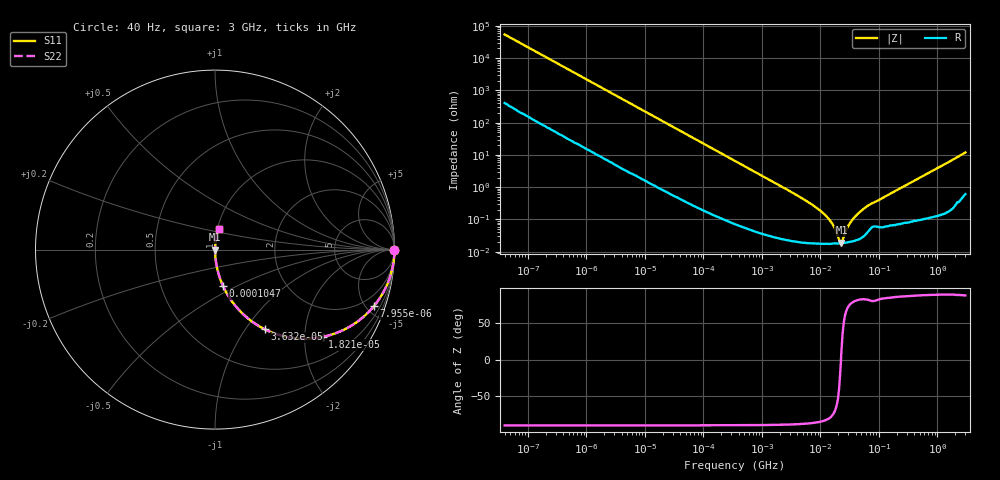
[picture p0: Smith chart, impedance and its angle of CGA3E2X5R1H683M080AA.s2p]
! S-parameter Generated by TDK Corporation
! Copyright(C) 2015 TDK Corporation.
! All Rights Reserved.
! TDK P/N: CGA3E2X5R1H683M080AA (Multilayer Ceramic Chip Capacitors)
! Property: C=68nF
! Size(LxWxT): 1.6x0.8x0.8mm, 0.063x0.031x0.031inches
! Model Type: s2p (Touchstone File Format Version 1.0)
! Frequency: DC=Yes Start=0.00004MHz Stop=3000MHz 396points Log-sweep
! Note: This model was converted from impedance.
! Model Generated on Jun. 23, 2015
! Hash(MD5):
! Port Assignments:
!  1 ---| |--- 2
! Applicable Conditions:
!  Temperature = 25 degC
!  DC Bias Voltage = 0 V
!  Small Signal Operation
! Terms and conditions regarding TDK Simulation Models
! (1)This simulation model is being provided solely for informational purposes. Please refer to the specifications of the products in terms of detailed characteristics of such products.
! (2)In no event shall TDK Corporation of any of its subsidiaries be liable for any loss or damage arising, directly or indirectly,
!  From any information contained in this simulation model, including, but not limited to loss or damages arising from any inaccuracies, omissions or errors in connection with such information.
! (3)Any and all copyrights on this simulation model are owned by TDK Corporation.
!  Duplication or redistribution of this simulation model without prior written permission from TDK Corporation is prohibited.
! (4)This simulation model is subject to any modification or change without any prior notice.
! (5)Neither TDK Corporation nor any of its subsidiaries shall make any warranty, express or implied,
!  Including but not limited to the correctness, implied warranties of merchantability and fitness for a particular purpose with respect to this simulation models.
! (6)The use of this simulation model shall be deemed to have consented to the terms and conditions hereof.
# MHz S MA R 50
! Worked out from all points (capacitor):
!   395 points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, 40 Hz to 3 GHz, reference 50 ohm
!   read as one part in series: C = 73.5 nF near 41.88 Hz
!   lowest |Z| = 19 mohm at 22.83 MHz (marker M1)
!   series resonance near 22.44 MHz, so ESL is about 680 pH
!   S11 on the Smith chart (normalised r, x): 40 Hz: open; 7.955 kHz: 1.04, -5.59; 18.21 kHz: 1.02, -2.45; 36.32 kHz: 1.01, -1.23; 104.7 kHz: 1.00, -0.43; 3 GHz: 1.01, +0.24
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4e-05  1 -0.1  0.001852 89.5  0.001852 89.5  1 -0.1
0.000834128  0.999 -2.2  0.03789 87.4  0.03789 87.4  0.999 -2.2
0.002889976  0.9907 -7.4  0.1294 82.2  0.1294 82.2  0.9907 -7.4
0.007954602  0.9393 -19.7  0.3363 69.9  0.3363 69.9  0.9393 -19.7
0.01739424  0.7856 -37.8  0.613 51.8  0.613 51.8  0.7856 -37.8
0.01821348  0.7716 -39.1  0.6304 50.5  0.6304 50.5  0.7716 -39.1
0.03632493  0.5226 -58.1  0.8486 31.5  0.8486 31.5  0.5226 -58.1
0.06026525  0.3479 -69.2  0.9348 20.4  0.9348 20.4  0.3479 -69.2
0.1046927  0.2098 -77.4  0.976 12.1  0.976 12.1  0.2098 -77.4
0.3464102  0.06526 -85.6  0.9972 3.7  0.9972 3.7  0.06526 -85.6
7.22376  0.002867 -86.2  0.9998 0.2  0.9998 0.2  0.002867 -86.2
10.93076  0.001616 -83.7  0.9998 0.1  0.9998 0.1  0.001616 -83.7
14.40706  0.0009554 -79.4  0.9998 0.1  0.9998 0.1  0.0009554 -79.4
17.31909  0.0005677 -71.3  0.9998 0.0  0.9998 0.0  0.0005677 -71.3
21.8003  0.0001946 -17.7  0.9998 0.0  0.9998 0.0  0.0001946 -17.7
22.82706  0.0001898 11.0  0.9998 -0.0  0.9998 -0.0  0.0001898 11.0
30.08671  0.0006505 72.1  0.9998 -0.0  0.9998 -0.0  0.0006505 72.1
41.52283  0.00138 80.3  0.9998 -0.1  0.9998 -0.1  0.00138 80.3
65.79027  0.002732 80.9  0.9996 -0.2  0.9996 -0.2  0.002732 80.9
150.6385  0.006067 83.6  0.9993 -0.3  0.9993 -0.3  0.006067 83.6
994.0817  0.03868 85.9  0.998 -2.2  0.998 -2.2  0.03868 85.9
3000  0.1181 80.3  0.987 -6.8  0.987 -6.8  0.1181 80.3
